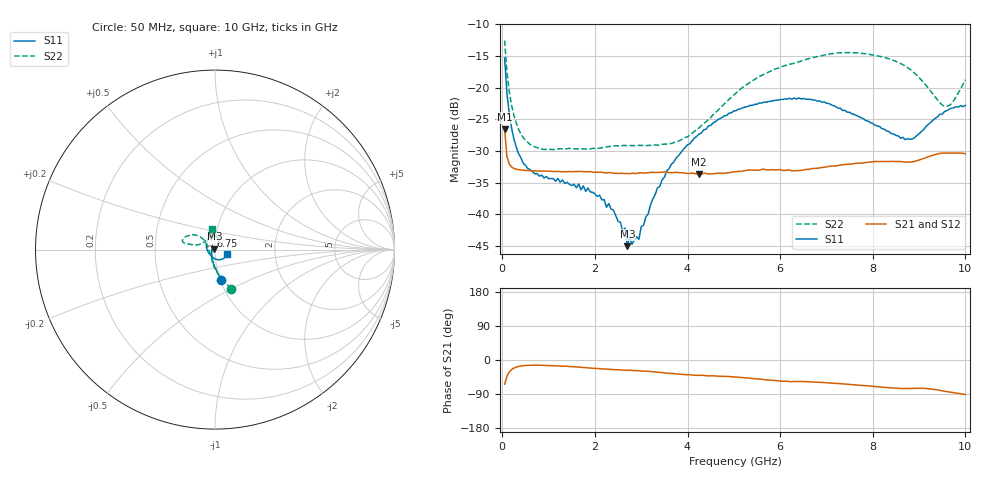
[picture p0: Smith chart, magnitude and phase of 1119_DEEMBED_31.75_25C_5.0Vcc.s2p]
!Hittite Microwave Corp.
!Digital Attenuator/PhaseShifter Rev 1.4.0
!Filename: C:\DATA\DATA\1119_DEEMBED_31.75_25C_5.0Vcc.s2p
!VNA ID: Agilent Technologies,N5224A,MY51441122,A.10.45.03
!Device type:
!2 Port Calibration.
!Temp(C): 25
!Lot Number:
!Serial Number:
!Operator:
!Misc:
!Attenuator:  31.750
# GHZ S DB R 50.0
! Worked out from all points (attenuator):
!   200 points, 50 MHz to 10 GHz, reference 50 ohm
!   highest |S21| = -26.62 dB at 50 MHz (marker M1); lowest = -33.7 dB at 4.25 GHz (marker M2)
!   lowest |S11| = -45.0 dB at 2.7 GHz (marker M3), VSWR 1.01, Z = 49.7 + j0.436 ohm
!   |S11| at or under -10 dB: start of sweep to end of sweep
!   |S22| runs from -29.8 to -12.6 dB; largest |S21 - S12| = 8.7e-05
!   S11 on the Smith chart (normalised r, x): 50 MHz: 1.01, -0.35; 6.75 GHz: 0.94, +0.14; 10 GHz: 1.15, -0.05
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0.05  -15.35 -78.5  -26.62 -63.9  -26.63 -63.9  -12.56 -67.6
0.1  -20.88 -93.0  -30.88 -43.3  -30.88 -43.3  -17.51 -84.0
0.2  -26.37 -109.2  -32.54 -25.3  -32.54 -25.3  -22.78 -100.6
0.45  -31.92 -136.0  -33.05 -15.1  -33.06 -15.2  -27.87 -121.4
0.85  -33.82 -160.5  -33.18 -14.0  -33.18 -14.0  -29.72 -135.0
1.75  -35.54 179.5  -33.28 -19.8  -33.29 -19.8  -29.68 -140.9
2.3  -38.32 163.5  -33.43 -24.2  -33.43 -24.2  -29.31 -149.4
2.65  -42.19 132.5  -33.59 -26.7  -33.59 -26.8  -29.14 -154.1
2.7  -45.05 128.2  -33.57 -27.1  -33.57 -27.1  -29.19 -154.6
2.75  -43.58 120.9  -33.60 -27.1  -33.61 -27.2  -29.15 -155.6
2.95  -43.97 94.1  -33.46 -28.4  -33.49 -28.5  -29.14 -160.3
3  -41.97 78.2  -33.47 -29.1  -33.49 -29.1  -29.13 -161.8
3.4  -35.64 65.3  -33.38 -32.5  -33.40 -32.5  -29.06 -173.9
3.65  -32.12 60.5  -33.47 -35.3  -33.46 -35.4  -28.82 176.9
4.25  -27.32 59.8  -33.67 -40.6  -33.69 -40.7  -26.37 151.9
5.05  -23.64 71.1  -33.30 -44.9  -33.30 -44.9  -20.83 138.5
6.7  -21.97 107.5  -32.79 -58.0  -32.81 -58.0  -15.27 153.8
6.75  -21.95 108.1  -32.77 -58.4  -32.78 -58.5  -15.19 154.4
8.35  -26.93 176.6  -31.69 -73.1  -31.68 -73.1  -15.45 168.1
8.85  -28.14 -133.6  -31.75 -74.9  -31.75 -74.9  -17.40 168.0
9.55  -23.78 -58.7  -30.34 -82.5  -30.35 -82.6  -22.92 138.1
10  -22.82 -18.9  -30.46 -91.2  -30.46 -91.2  -18.77 98.2
